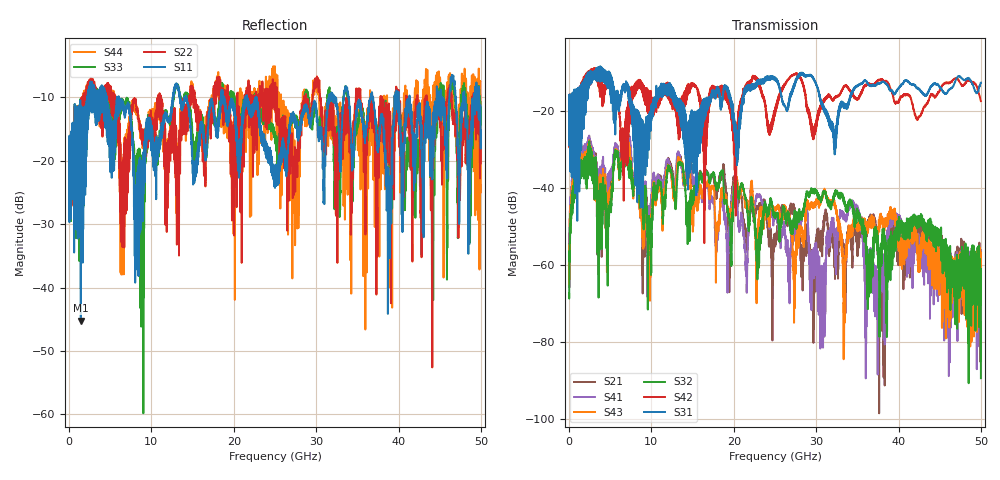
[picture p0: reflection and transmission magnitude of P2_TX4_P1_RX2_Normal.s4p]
!Keysight Technologies,N5225B,MY57041031,A.13.20.10
!Date: Friday, May 31, 2019 11:16:30
!Correction: S11(Full 4 Port(1,2,3,4))
!S12(Full 4 Port(1,2,3,4))
!S13(Full 4 Port(1,2,3,4))
!S14(Full 4 Port(1,2,3,4))
!S21(Full 4 Port(1,2,3,4))
!S22(Full 4 Port(1,2,3,4))
!S23(Full 4 Port(1,2,3,4))
!S24(Full 4 Port(1,2,3,4))
!S31(Full 4 Port(1,2,3,4))
!S32(Full 4 Port(1,2,3,4))
!S33(Full 4 Port(1,2,3,4))
!S34(Full 4 Port(1,2,3,4))
!S41(Full 4 Port(1,2,3,4))
!S42(Full 4 Port(1,2,3,4))
!S43(Full 4 Port(1,2,3,4))
!S44(Full 4 Port(1,2,3,4))
!S4P File: Measurements: <S11,S12,S13,S14>,
!<S21,S22,S23,S24>,
!<S31,S32,S33,S34>,
!<S41,S42,S43,S44>:
# Hz S  dB  R 50.0
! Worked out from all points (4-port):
!   5000 points, 10 MHz to 50 GHz, reference 50 ohm
!   strongest paths, dB at 10 MHz, 12.51 GHz, 25.01 GHz, 37.51 GHz, 50 GHz:
!     S31: -19.3, -14.2, -11.3, -12.8, -12.6
!     S42: -19.3, -16.3, -19.4, -11.9, -17.3
!     S32: -67.3, -36.9, -47.6, -53.7, -89.3
!     S43: -64.9, -38.6, -45.2, -52.1, -65.3
!     S41: -65.6, -37.8, -47.0, -74.3, -74.1
!     S21: -60.4, -35.3, -52.3, -56.6, -61.5
!   lowest |S11| = -45.2 dB at 1.43 GHz (marker M1), VSWR 1.01, Z = 49.5 + j0.131 ohm
!   |S11| at or under -10 dB: 6.023 GHz to 12.61 GHz (6.592 GHz wide, 70.7 % of centre); 14.2 GHz to 18.43 GHz (4.229 GHz wide, 25.9 % of centre); 22.71 GHz to 31.52 GHz (8.807 GHz wide, 32.5 % of centre)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
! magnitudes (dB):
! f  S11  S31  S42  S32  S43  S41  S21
! 10 MHz  -19.0  -19.3  -19.3  -67.3  -64.9  -65.6  -60.4
! 1.43 GHz  -45.2  -26.8  -17.1  -33.2  -31.8  -30.0  -31.6
! 29.61 GHz  -11.8  -11.5  -27.2  -41.0  -44.7  -59.0  -61.5
! 36.84 GHz  -10.1  -13.2  -13.2  -60.3  -48.2  -60.5  -47.4
! 38.26 GHz  -15.2  -12.4  -12.2  -51.9  -49.6  -57.0  -75.4
! 42.78 GHz  -14.4  -14.9  -20.5  -48.9  -55.9  -56.9  -50.5
! 50 GHz  -15.3  -12.6  -17.3  -89.3  -65.3  -74.1  -61.5
